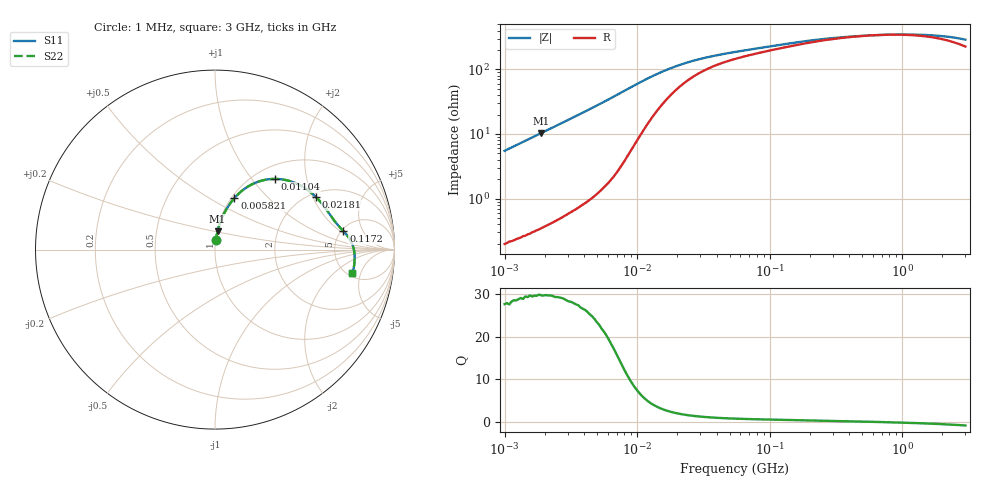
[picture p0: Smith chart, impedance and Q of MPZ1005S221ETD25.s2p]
! S-parameter Generated by TDK Corporation
! Copyright(C) 2016 TDK Corporation.
! All Rights Reserved.
! TDK P/N: MPZ1005S221ETD25 (Chip Beads)
! Property: |Z|=220¶ at 100MHz
! Size(LxWxT): 1x0.5x0.5mm, 0.039x0.02x0.02inches
! Model Type: s2p (Touchstone File Format Version 1.0)
! Frequency: DC=Yes Start=1MHz Stop=3000MHz 202points Log-sweep
! Note: This model was converted from impedance.
! Model Generated on May. 16, 2016
! Hash(MD5):
! Port Assignments:
!  1 ---@@@--- 2
! Applicable Conditions:
!  Temperature = 25 degC
!  DC Bias Current = 0 A
!  Small Signal Operation
! Terms and conditions regarding TDK Simulation Models
! (1)This simulation model is being provided solely for informational purposes. Please refer to the specifications of the products in terms of detailed characteristics of such products.
! (2)In no event shall TDK Corporation of any of its subsidiaries be liable for any loss or damage arising, directly or indirectly,
!  From any information contained in this simulation model, including, but not limited to loss or damages arising from any inaccuracies, omissions or errors in connection with such information.
! (3)Any and all copyrights on this simulation model are owned by TDK Corporation.
!  Duplication or redistribution of this simulation model without prior written permission from TDK Corporation is prohibited.
! (4)This simulation model is subject to any modification or change without any prior notice.
! (5)Neither TDK Corporation nor any of its subsidiaries shall make any warranty, express or implied,
!  Including but not limited to the correctness, implied warranties of merchantability and fitness for a particular purpose with respect to this simulation models.
! (6)The use of this simulation model shall be deemed to have consented to the terms and conditions hereof.
# MHz S MA R 50
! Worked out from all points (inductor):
!   201 points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, 1 MHz to 3 GHz, reference 50 ohm
!   read as one part in series: L = 871 nH near 1.041 MHz
!   highest Q = 29.7 at 1.897 MHz (marker M1), where L = 869 nH
!   self-resonance near 702.7 MHz
!   S11 on the Smith chart (normalised r, x): 1 MHz: 1.00, +0.11; 5.821 MHz: 1.03, +0.65; 11.04 MHz: 1.22, +1.31; 21.81 MHz: 2.16, +2.11; 117.2 MHz: 5.20, +2.26; 3 GHz: 5.52, -3.59
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1  0.05465 84.8  0.9965 -3.1  0.9965 -3.1  0.05465 84.8
1.897447  0.1027 82.2  0.9913 -5.9  0.9913 -5.9  0.1027 82.2
2.720446  0.1463 79.6  0.9842 -8.4  0.9842 -8.4  0.1463 79.6
3.900413  0.2079 75.9  0.9703 -12.0  0.9703 -12.0  0.2079 75.9
5.820586  0.306 69.4  0.9372 -17.8  0.9372 -17.8  0.306 69.4
7.703107  0.396 62.4  0.889 -23.3  0.889 -23.3  0.396 62.4
9.410094  0.4646 55.8  0.8331 -27.5  0.8331 -27.5  0.4646 55.8
11.04425  0.5149 49.9  0.7759 -30.5  0.7759 -30.5  0.5149 49.9
12.45355  0.5472 45.4  0.7284 -32.3  0.7284 -32.3  0.5472 45.4
14.61624  0.5817 39.6  0.6644 -33.9  0.6644 -33.9  0.5817 39.6
17.85516  0.6128 33.0  0.5897 -34.5  0.5897 -34.5  0.6128 33.0
21.81181  0.634 27.5  0.5265 -33.8  0.5265 -33.8  0.634 27.5
32.54976  0.6608 19.5  0.4367 -30.3  0.4367 -30.3  0.6608 19.5
54.77226  0.6855 13.3  0.3685 -25.4  0.3685 -25.4  0.6855 13.3
117.1891  0.7226 8.3  0.3031 -20.0  0.3031 -20.0  0.7226 8.3
213.6344  0.748 5.2  0.2639 -14.9  0.2639 -14.9  0.748 5.2
405.36  0.7651 2.4  0.2377 -7.6  0.2377 -7.6  0.7651 2.4
800.5644  0.7756 -0.6  0.2246 2.0  0.2246 2.0  0.7756 -0.6
1243.477  0.7791 -2.9  0.2253 10.0  0.2253 10.0  0.7791 -2.9
1712.864  0.7803 -4.9  0.2321 16.6  0.2321 16.6  0.7803 -4.9
2266.846  0.7802 -7.0  0.2449 22.9  0.2449 22.9  0.7802 -7.0
3000  0.7756 -9.6  0.2686 28.8  0.2686 28.8  0.7756 -9.6
